ORGANIZATION_BLOCK "Hardware Interrupt 7"
TITLE =
VERSION : 0.1


VAR_TEMP
  OB47_EV_CLASS : BYTE ;	//Bits 0-3 = 1 (Coming event), Bits 4-7 = 1 (Event class 1)
  OB47_STRT_INF : BYTE ;	//16#41/42/43/44 (Interrupt 1/2/3/4)
  OB47_PRIORITY : BYTE ;	//23 (Priority of 1 is lowest)
  OB47_OB_NUMBR : BYTE ;	//47 (Organization block 47, OB47)
  OB47_RESERVED_1 : BYTE ;	//Reserved for system
  OB47_RESERVED_2 : BYTE ;	//Reserved for system
  OB47_MDL_ADDR : WORD ;	//Base address of module initiating interrupt
  OB47_POINT_ADDR : DWORD ;	//Address of interrupt point on module
  OB47_DATE_TIME : DATE_AND_TIME ;	//Date and time OB47 started
END_VAR
BEGIN
END_ORGANIZATION_BLOCK

